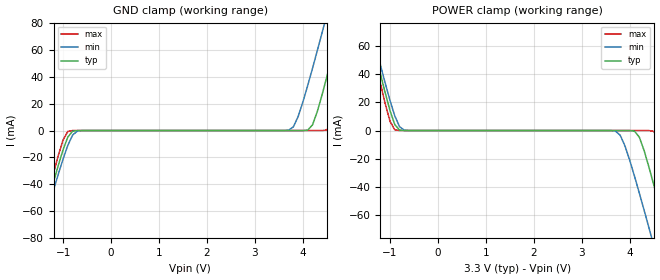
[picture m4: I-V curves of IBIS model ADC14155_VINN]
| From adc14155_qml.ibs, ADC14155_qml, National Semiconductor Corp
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|   Model of Differential Inputs ADC14155_VINN
[Model]   ADC14155_VINN
Model_type Input
Polarity Inverting
Vinh=2.0
Vinl=1.0
C_comp   776.6f   764.4f   787.6f
[Temperature Range] 25   85   -40
[Voltage Range]   3.3   3.0   3.6
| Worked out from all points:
|   GND clamp passes 1 mA (typ) near -0.81 V on its own axis
|   POWER clamp passes 1 mA (typ) near -0.82 V on its own axis
[GND Clamp]
|V(groundclamp)   I(typ)   I(min)   I(max)
-3.3V     -322.4mA   -312.6mA   -335.1mA
-1.5V     -77.49mA   -81.34mA   -73.54mA
-1.1V     -25.94mA   -32.53mA   -18.6mA
-900mV    -4.742mA   -10.9mA    -604uA
-600mV    -278.4nA   -17.67uA   -369.6pA
3.7V      84.77pA    241.1uA    8.991pA
3.9V      166.1nA    10.36mA    9.951pA
4.2V      4.188mA    46.42mA    221.4pA
4.5V      40.21mA    86.59mA    437.8uA
4.8V      82.74mA    127.8mA    33.34mA
5.1V      126.5mA    169.5mA    78.82mA
6.5V      334.4mA    366.6mA    299.9mA
[POWER Clamp]
|V(PowerClamp)   I(typ)   I(min)   I(max)
-3.3V     349.4mA    338.3mA    315.9mA
-1.5V     82.74mA    86.59mA    78.82mA
-1.4V     68.37mA    73.03mA    63.43mA
-900mV    4.188mA    10.36mA    437.8uA
-700mV    7.783uA    241.1uA    28.92nA
3.7V      -141.7pA   -368.4uA   -7.681pA
3.9V      -278.4nA   -10.9mA    -8.642pA
4.2V      -4.742mA   -44.39mA   -369.6pA
4.5V      -38.39mA   -81.34mA   -604uA
4.8V      -77.49mA   -119.2mA   -31.74mA
5.1V      -117.7mA   -157.5mA   -73.54mA
6.5V      -308.6mA   -312.6mA   -276.5mA
